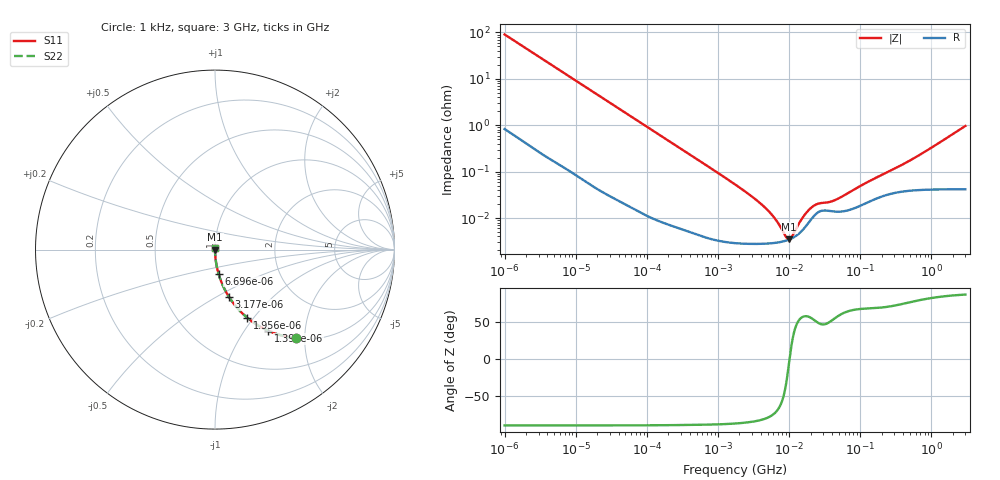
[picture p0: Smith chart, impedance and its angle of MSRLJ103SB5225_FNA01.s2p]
! MSRLJ103SB5225_FNA01  S-PARAMETER MODEL  ( Standard Model )
! Model Generated by TAIYO YUDEN Corporation (http://www.ty-top.com)
! Version 2.0
! TAIYO YUDEN Control No. 230320
! Copyright(c) 2013 TAIYO YUDEN CO.,LTD. All Rights Reserved.
! Product Description (link to TY-COMPAS)
! https://ds.yuden.co.jp/TYCOMPAS/or/detail?pn=MSRLJ103SB5225MFNA01&u=M
! Products Name : Multilayer Ceramic Capacitors
! Characteristics :
!  Capacitance : 2.2 [uF] , Rated Voltage : 6.3 [V] , TCC : X5R
!  Case Size : 0.52 x 1.0 / 0.02 x 0.039 [mm/inch] , Thickness : 0.3 / 0.012 [mm/inch]
!  (Conditions: Temperature = 25 [degC] , DC Bias Voltage = 0 [V])
! External Node Assignments :
!  1  o---| |---o  2
! GND o---------o GND
! Frequency Range : 1kHz  -  3GHz  [ 401 STEP ]
# MHZ S RI R 50
! Freq[MHz].  S11 Real  S11 Imag  S21 Real  S21 Imag  S12 Real  S12 Imag  S22 Real  S22 Imag
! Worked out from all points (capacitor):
!   401 points, 1 kHz to 3 GHz, reference 50 ohm
!   read as one part in series: C = 1.75 uF near 1.077 kHz
!   lowest |Z| = 3.45 mohm at 9.991 MHz (marker M1)
!   series resonance near 10.12 MHz, so ESL is about 140 pH
!   S11 on the Smith chart (normalised r, x): 1 kHz: 1.02, -1.81; 1.399 kHz: 1.01, -1.30; 1.956 kHz: 1.01, -0.93; 3.177 kHz: 1.01, -0.57; 6.696 kHz: 1.00, -0.27; 3 GHz: 1.00, +0.02
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0.001  0.4509 -0.493  0.5491 0.493  0.5491 0.493  0.4509 -0.493
0.001399  0.2978 -0.4528  0.7022 0.4528  0.7022 0.4528  0.2978 -0.4528
0.001956  0.1797 -0.3795  0.8203 0.3795  0.8203 0.3795  0.1797 -0.3795
0.003177  0.078 -0.2638  0.922 0.2638  0.922 0.2638  0.078 -0.2638
0.006696  0.0195 -0.1338  0.9805 0.1338  0.9805 0.1338  0.0195 -0.1338
0.01216  0.00635 -0.075  0.9937 0.075  0.9937 0.075  0.00635 -0.075
0.033275  0.00104 -0.0277  0.999 0.0277  0.999 0.0277  0.00104 -0.0277
0.147855  0.000125 -0.00629  0.9999 0.00629  0.9999 0.00629  0.000125 -0.00629
1.732051  2.9e-05 -0.00053  1 0.00053  1 0.00053  2.9e-05 -0.00053
3.651041  2.77e-05 -0.000227  1 0.000227  1 0.000227  2.77e-05 -0.000227
6.153411  2.9e-05 -9.83e-05  1 9.83e-05  1 9.83e-05  2.9e-05 -9.83e-05
6.881678  2.97e-05 -7.52e-05  1 7.52e-05  1 7.52e-05  2.97e-05 -7.52e-05
9.991309  3.44e-05 -2.42e-06  1 2.42e-06  1 2.42e-06  3.44e-05 -2.42e-06
15.05716  5.28e-05 8.02e-05  0.9999 -8.02e-05  0.9999 -8.02e-05  5.28e-05 8.02e-05
21.06097  9.97e-05 0.000142  0.9999 -0.000142  0.9999 -0.000142  9.97e-05 0.000142
25.37713  0.000132 0.000154  0.9999 -0.000154  0.9999 -0.000154  0.000132 0.000154
36.84432  0.000142 0.000171  0.9999 -0.000171  0.9999 -0.000171  0.000142 0.000171
46.08157  0.000137 0.00021  0.9999 -0.00021  0.9999 -0.00021  0.000137 0.00021
121.4899  0.000211 0.000538  0.9998 -0.000538  0.9998 -0.000538  0.000211 0.000538
256.0921  0.000327 0.000965  0.9997 -0.000965  0.9997 -0.000965  0.000327 0.000965
650.4536  0.000404 0.00216  0.9996 -0.00216  0.9996 -0.00216  0.000404 0.00216
3000  0.00051 0.00964  0.9995 -0.00964  0.9995 -0.00964  0.00051 0.00964
